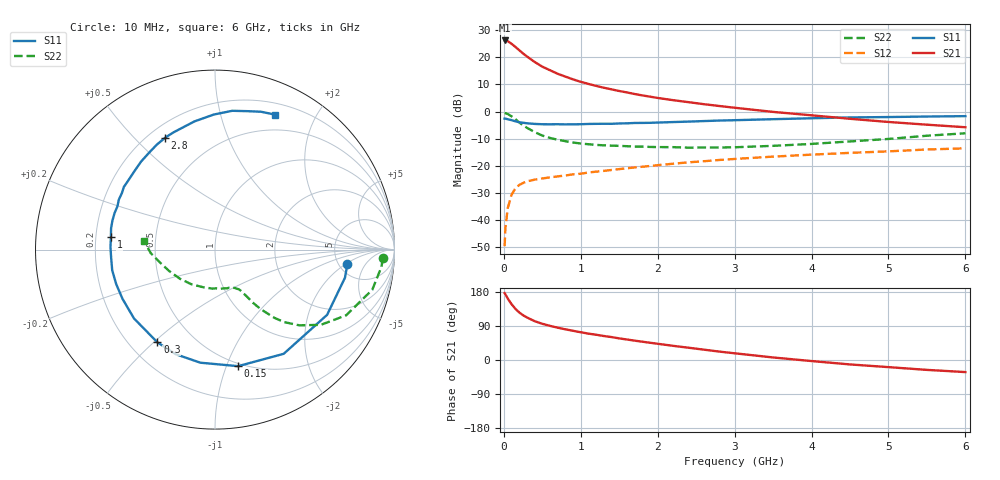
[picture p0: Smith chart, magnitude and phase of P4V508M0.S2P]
! SIEMENS Small Signal Semiconductors
! BFP182
! Si NPN RF Bipolar Junction Transistor in SOT143
! VCE = 0.5 V  IC = 8 mA
! Common Emitter S-Parameters:  March  1996
# GHz  S  MA  R  50
!  f  S11  S21  S12  S22
! GHz  MAG  ANG  MAG  ANG  MAG  ANG  MAG  ANG
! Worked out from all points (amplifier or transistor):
!   36 points, 10 MHz to 6 GHz, reference 50 ohm
!   highest |S21| = 26.2 dB at 10 MHz (marker M1)
!   |S21| within 3 dB of that: start of sweep to 176 MHz
!   unconditionally stable (mu >= 1): 770 MHz to end of sweep
!   at 250 MHz: K = 0.40, MSG = 23.9 dB, |S12| = -26.3 dB
!   at 1.4 GHz: K = 1.39, MAG = 11.1 dB, |S12| = -21.5 dB
!   at 6 GHz: K = 1.33, MAG = 0.5 dB, |S12| = -13.6 dB
!   S11 on the Smith chart (normalised r, x): 10 MHz: 5.95, -2.15; 150 MHz: 0.48, -1.10; 300 MHz: 0.31, -0.51; 1 GHz: 0.26, +0.06; 2.8 GHz: 0.26, +0.62; 6 GHz: 0.32, +1.49
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0.01  0.7419 -6.3  20.46 176.7  0.0033 86.5  0.9367 -2.9
0.02  0.7409 -12.2  20.43 173.3  0.007 83.4  0.9323 -5.9
0.05  0.7227 -30.2  19.88 162.5  0.0164 75.2  0.9045 -14.3
0.1  0.6954 -56.6  17.77 147.4  0.0293 62.0  0.8174 -26.6
0.15  0.662 -78.8  15.58 135.2  0.0384 53.1  0.7236 -35.4
0.2  0.6354 -97.4  13.54 125.5  0.0443 46.8  0.6317 -41.9
0.25  0.6225 -110.7  11.75 118.1  0.0482 41.9  0.5578 -46.4
0.3  0.6081 -121.9  10.39 112.3  0.0516 38.9  0.5032 -49.0
0.4  0.5923 -139.6  8.218 102.5  0.0556 35.6  0.4178 -52.5
0.5  0.5838 -151.9  6.728 95.5  0.0584 33.1  0.3611 -54.6
0.6  0.5831 -160.8  5.778 90.1  0.0612 32.8  0.3265 -55.5
0.7  0.5842 -168.6  4.971 85.3  0.0639 32.8  0.3028 -56.4
1  0.5842 173.1  3.532 73.2  0.0714 33.5  0.2577 -59.1
1.1  0.5911 168.4  3.234 69.6  0.0753 34.0  0.2499 -60.7
1.5  0.6038 152.6  2.394 57.0  0.0868 34.5  0.233 -66.3
1.8  0.6175 142.0  1.986 48.3  0.0961 34.5  0.226 -72.6
2.2  0.6405 130.0  1.622 37.4  0.1092 32.9  0.2208 -82.4
2.8  0.6827 114.0  1.267 22.2  0.128 29.5  0.2173 -100.7
3.5  0.7234 99.1  0.986 6.7  0.1476 24.5  0.2334 -124.0
4.5  0.7793 82.9  0.736 -11.7  0.1733 16.7  0.2814 -154.7
5.5  0.8098 71.5  0.573 -26.1  0.1999 9.2  0.3587 -176.9
6  0.8234 65.9  0.514 -31.9  0.2101 4.4  0.3978 173.1
